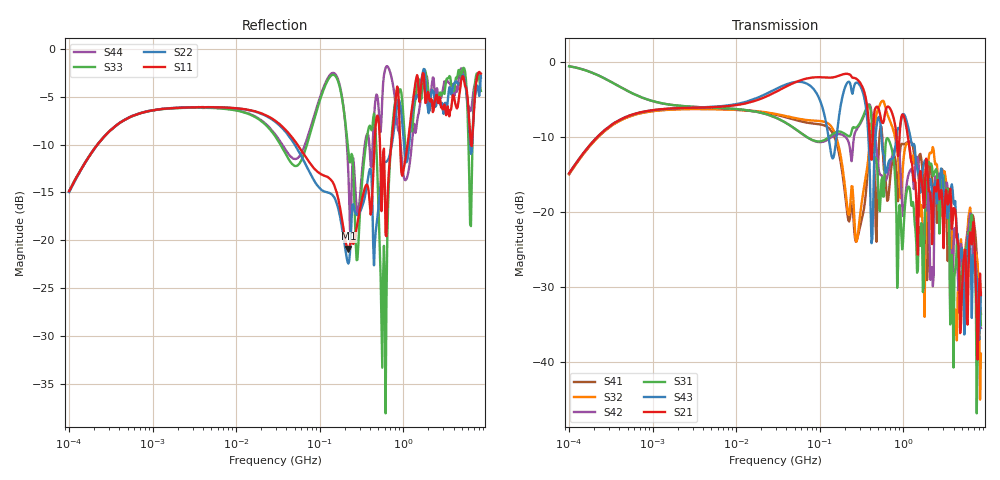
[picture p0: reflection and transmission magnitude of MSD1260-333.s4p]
# MHz S MA R 50
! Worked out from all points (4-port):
!   498 points, 100 kHz to 8.5 GHz, reference 50 ohm
!   strongest paths, dB at 100 kHz, 1.698 MHz, 29.49 MHz, 500.7 MHz, 8.5 GHz:
!     S21: -14.8, -6.2, -4.0, -6.1, -31.1
!     S43: -14.9, -6.2, -3.6, -7.4, -30.8
!     S31: -0.6, -5.7, -7.4, -16.3, -35.1
!     S42: -0.5, -5.7, -7.4, -13.8, -35.5
!     S32: -15.0, -6.3, -6.9, -6.3, -38.9
!     S41: -15.0, -6.3, -7.0, -13.6, -33.6
!   lowest |S11| = -20.9 dB at 220 MHz (marker M1), VSWR 1.20, Z = 58.4 - j5 ohm
!   |S11| at or under -10 dB: 53.97 MHz to 453 MHz (399 MHz wide, 157 % of centre); 526.2 MHz to 719 MHz (192.9 MHz wide, 31 % of centre); 919.3 MHz to 1.127 GHz (208 MHz wide, 20.3 % of centre)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
0.1  0.1804 67.2  0.181 67.4  0.9386 -10.3  0.1784 -113.0
     0.181 67.4  0.1785 67.3  0.1784 -112.9  0.9403 -10.3
     0.9386 -10.3  0.1784 -112.9  0.1789 67.2  0.1807 67.1
     0.1784 -113.0  0.9403 -10.3  0.1807 67.1  0.1811 67.4
220.0307  0.09025 -28.1  0.8336 -44.7  0.3212 60.7  0.08808 -32.8
          0.8336 -44.7  0.07554 -16.0  0.09636 -26.1  0.2955 56.1
          0.3212 60.7  0.09636 -26.1  0.2914 -85.9  0.7392 -30.1
          0.08808 -32.8  0.2955 56.1  0.7392 -30.1  0.2265 -92.0
587.4518  0.3009 -67.6  0.4067 -81.8  0.1266 -27.2  0.1908 -56.2
          0.4067 -81.8  0.2539 -22.1  0.5431 -65.4  0.1637 151.1
          0.1266 -27.2  0.5431 -65.4  0.09352 -61.2  0.2368 -94.7
          0.1908 -56.2  0.1637 151.1  0.2368 -94.7  0.7258 -48.5
827.4608  0.5959 -72.9  0.3242 -137.2  0.09719 174.5  0.1857 -79.0
          0.3242 -137.2  0.4754 -60.2  0.2855 -156.0  0.2816 -50.6
          0.09719 174.5  0.2855 -156.0  0.5718 -62.9  0.3145 -70.2
          0.1857 -79.0  0.2816 -50.6  0.3145 -70.2  0.453 -145.1
1840.304  0.5207 -169.2  0.184 170.7  0.1117 -116.1  0.105 130.2
          0.184 170.7  0.7017 -173.3  0.06048 -66.1  0.1011 148.2
          0.1117 -116.1  0.06048 -66.1  0.7659 -165.8  0.2221 147.5
          0.105 130.2  0.1011 148.2  0.2221 147.5  0.7051 -152.3
2972.863  0.4831 83.9  0.09968 -127.2  0.1735 42.0  0.1884 47.2
          0.09968 -127.2  0.481 82.2  0.1656 46.8  0.1635 59.3
          0.1735 42.0  0.1656 46.8  0.5896 78.1  0.167 -21.6
          0.1884 47.2  0.1635 59.3  0.167 -21.6  0.6064 84.8
8500  0.7424 -54.1  0.02784 -108.5  0.01752 -89.1  0.02093 -121.0
      0.02784 -108.5  0.7248 -41.4  0.01129 -16.7  0.01673 -88.8
      0.01752 -89.1  0.01129 -16.7  0.6019 -48.7  0.02869 -94.2
      0.02093 -121.0  0.01673 -88.8  0.02869 -94.2  0.7064 -52.4
